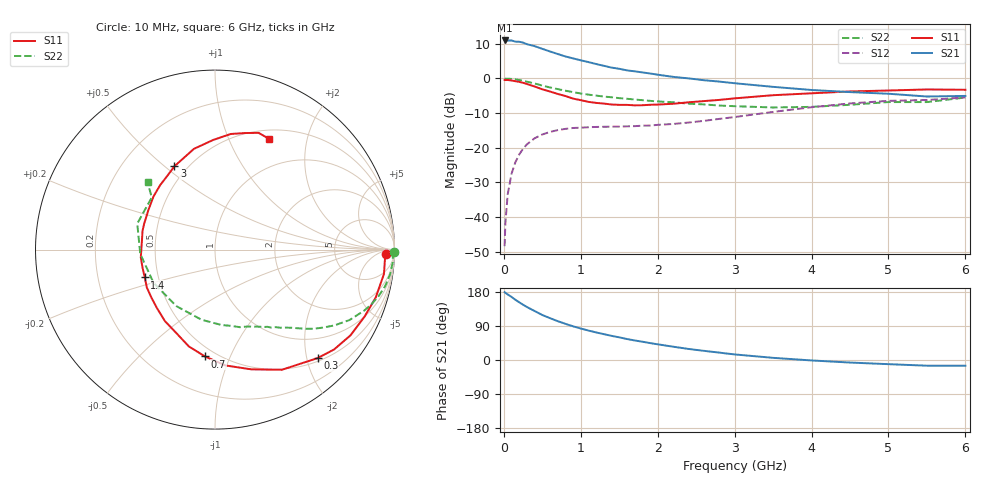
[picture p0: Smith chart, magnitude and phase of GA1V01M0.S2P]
! Infineon Technologies  Discrete & RF Semiconductors
! BF775
! Si NPN RF Bipolar Junction Transistor in SOT23
! VCE = 1 V  IC = 1 mA
! Common Emitter S-Parameters:  May  1996
# GHz  S  MA  R  50
!  f  S11  S21  S12  S22
! GHz  MAG  ANG  MAG  ANG  MAG  ANG  MAG  ANG
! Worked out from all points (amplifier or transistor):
!   36 points, 10 MHz to 6 GHz, reference 50 ohm
!   highest |S21| = 11.0 dB at 10 MHz (marker M1)
!   |S21| within 3 dB of that: start of sweep to 576.5 MHz
!   unconditionally stable (mu >= 1): 1.342 GHz to end of sweep
!   at 250 MHz: K = 0.21, MSG = 15.3 dB, |S12| = -20.3 dB
!   at 1.4 GHz: K = 1.04, MAG = 7.3 dB, |S12| = -13.9 dB
!   at 6 GHz: K = 1.09, MAG = -1.6 dB, |S12| = -5.5 dB
!   S11 on the Smith chart (normalised r, x): 10 MHz: 31, -18; 300 MHz: 0.56, -2.20; 700 MHz: 0.44, -0.81; 1.4 GHz: 0.42, -0.16; 3 GHz: 0.43, +0.54; 6 GHz: 0.61, +1.42
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0.01  0.9532 -1.6  3.537 179.0  0.0038 86.4  0.9999 -0.8
0.02  0.9484 -3.2  3.464 177.1  0.0081 86.8  0.9912 -1.6
0.05  0.9511 -8.2  3.532 173.1  0.0212 85.0  0.993 -4.0
0.1  0.9344 -16.6  3.535 166.4  0.0421 79.8  0.9848 -8.1
0.15  0.9132 -24.1  3.399 158.9  0.0618 74.5  0.9701 -12.0
0.2  0.8934 -32.3  3.391 152.3  0.0801 69.7  0.9494 -15.6
0.25  0.8659 -40.0  3.288 145.9  0.0968 65.1  0.9238 -19.2
0.3  0.832 -46.6  3.127 139.8  0.1119 61.1  0.8984 -22.2
0.4  0.7663 -60.9  2.928 129.3  0.1371 53.8  0.8463 -27.6
0.5  0.6974 -73.1  2.678 118.7  0.1555 47.4  0.7894 -32.3
0.7  0.5981 -95.3  2.256 102.5  0.1798 38.1  0.7025 -38.9
0.9  0.512 -115.0  1.949 88.9  0.193 32.1  0.6352 -43.6
1.1  0.4596 -134.6  1.723 77.7  0.1978 28.3  0.5846 -48.0
1.4  0.421 -158.4  1.435 63.7  0.2016 25.2  0.5356 -54.2
1.7  0.4097 178.0  1.269 51.6  0.205 25.7  0.4962 -60.0
2.2  0.4316 149.3  1.055 35.1  0.2204 28.7  0.454 -72.2
3  0.5163 116.0  0.854 14.7  0.2775 32.0  0.3981 -100.8
3.5  0.5735 101.8  0.757 5.7  0.3289 30.1  0.3815 -124.5
4.5  0.6499 82.3  0.636 -6.7  0.4362 19.3  0.4172 -176.7
5  0.6705 75.6  0.602 -11.0  0.4755 12.2  0.4566 161.5
5.5  0.6943 69.5  0.549 -15.0  0.4891 4.4  0.4565 140.5
6  0.6868 64.0  0.56 -15.1  0.5329 0.2  0.5312 135.0
